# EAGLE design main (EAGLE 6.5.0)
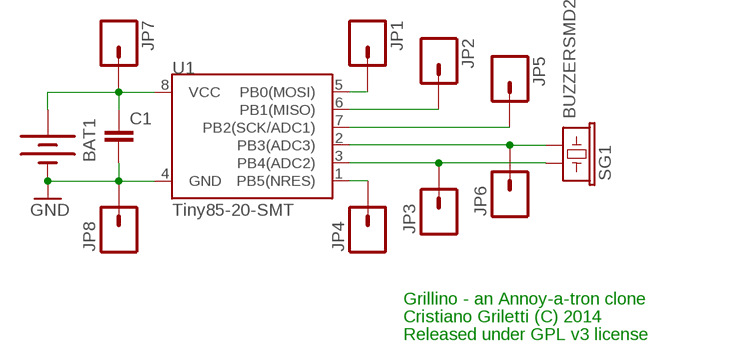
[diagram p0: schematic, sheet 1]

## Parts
BAT1  BATTERYFOB  [BATTERY_20MM_PTH_COMPACT]
C1  CAP0805  [0805]
JP1  M01SMD-4.5X1.5  [PAD-1.5X4.5]
JP2  M01SMD-4.5X1.5  [PAD-1.5X4.5]
JP3  M01SMD-4.5X1.5  [PAD-1.5X4.5]
JP4  M01SMD-4.5X1.5  [PAD-1.5X4.5]
JP5  M01SMD-4.5X1.5  [PAD-1.5X4.5]
JP6  M01SMD-4.5X1.5  [PAD-1.5X4.5]
JP7  M01SMD-4.5X1.5  [PAD-1.5X4.5]
JP8  M01SMD-4.5X1.5  [PAD-1.5X4.5]
SG1  BUZZERSMD2  [BUZZER-CCV]
U1  Tiny85-20-SMT  ATTINY45TINY85-20-SMT  [SO08-EIAJ]

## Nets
GND: BAT1.2(-) C1.2 JP8.P$1 U1.4(GND)
N$2: BAT1.1(+) C1.1 JP7.P$1 U1.8(VCC)
N$3: JP6.P$1 SG1.- U1.2(PB3(ADC3))
N$4: JP5.P$1 U1.7(PB2(SCK/ADC1))
N$5: JP1.P$1 U1.5(PB0(MOSI))
N$6: JP2.P$1 U1.6(PB1(MISO))
N$7: JP3.P$1 SG1.+ U1.3(PB4(ADC2))
N$8: JP4.P$1 U1.1(PB5(NRES))

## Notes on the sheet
- Grillino - an Annoy-a-tron clone
- Cristiano Griletti (C) 2014
- Released under GPL v3 license

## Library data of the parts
BAT1 = SparkFun-Electromechanical:BATTERY: Battery Holders
C1 = SparkFun-Passives:CAP: Capacitor
JP1-JP8 = SparkFun-Connectors:M01: Header 1
SG1 = SparkFun-Electromechanical:BUZZER: Buzzer 12mm
U1 = SparkFun-DigitalIC:ATTINY45: Atmel 8-pin 2/4/8kB flash uC; PROD_ID: IC-09092

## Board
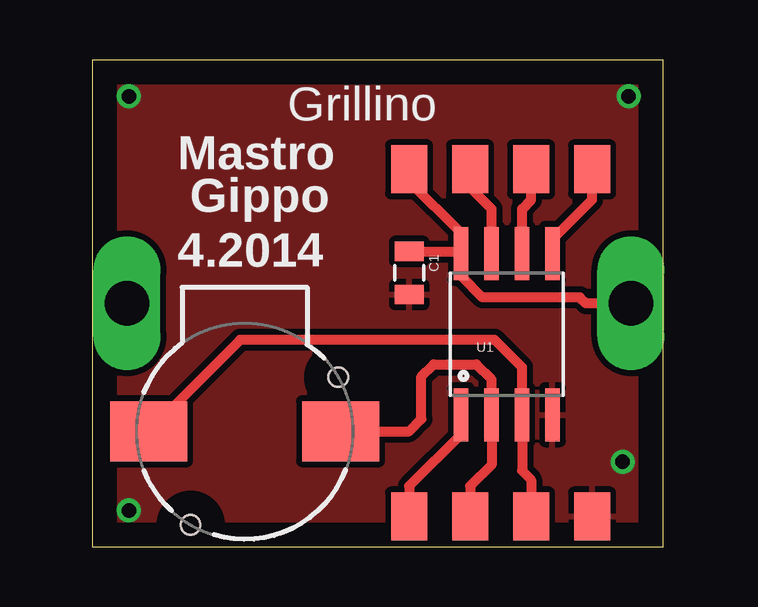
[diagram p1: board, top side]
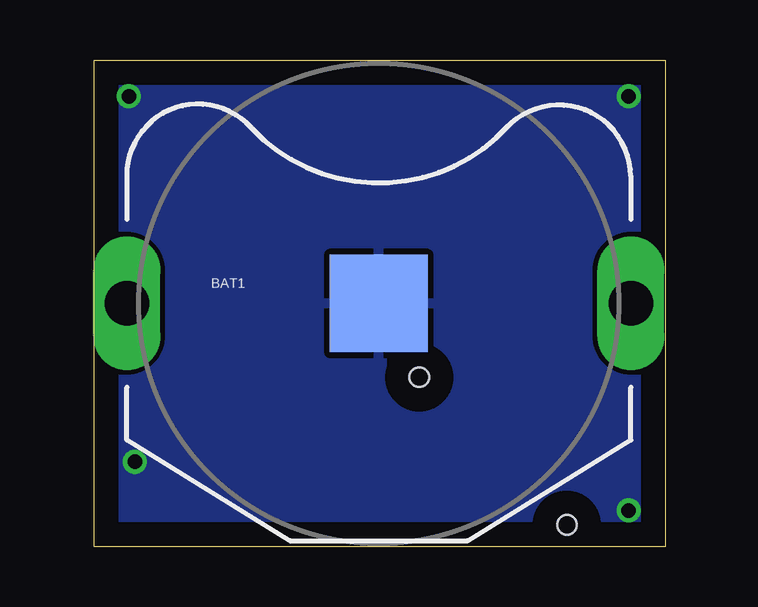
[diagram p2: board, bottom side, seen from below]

Size 23.8 x 20.31 mm. Coordinates in mm from the lower left corner, seen from the top.
Outline: 0,0 23.8,0 23.8,20.31 0,20.31 0,0
Copper layers (1*16): Top 0.035mm / dielectric 1.5mm / Bottom 0.035mm
Design rules "default": minimum track width 10mil, minimum drill 24mil, track to track 8mil, track to pad 8mil, pad to pad 8mil, via to via 8mil, smd to smd 8mil, copper to edge 40mil, drill to drill 8mil, minimum pad ring 10mil, minimum via ring 8mil, stop-mask expansion 4mil, vias tented up to drill 0mil, thermal gap 10mil

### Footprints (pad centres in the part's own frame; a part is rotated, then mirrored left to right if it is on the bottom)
BATTERY_20MM_PTH_COMPACT = drill 1.854 long: 1 -10.5,0; 3 10.5,0 | smd 4.064 x 4.064: 2 0,0
0805 = smd 0.8 x 1.2: 1 -0.9,0; 2 0.9,0
PAD-1.5X4.5 = smd 1.5 x 2: P$1 0,0
BUZZER-CCV = smd 3.2 x 2.5: + 4,0; - -4,0 | hole 0.8: -3.9,-2.25; 2.25,3.9
SO08-EIAJ = smd 0.61 x 2.21: 1 -1.905,-3.378; 2 -0.635,-3.378; 3 0.635,-3.378; 4 1.905,-3.378; 5 1.905,3.353; 6 0.635,3.353; 7 -0.635,3.353; 8 -1.905,3.353

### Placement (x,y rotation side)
BAT1  11.94,10.16 0 bottom
C1  13.21,11.43 270 top
JP1  20.83,15.75 0 top
JP2  18.29,15.75 0 top
JP3  18.29,1.27 0 top
JP4  13.21,1.27 0 top
JP5  15.75,15.75 0 top
JP6  15.75,1.27 0 top
JP7  13.21,15.75 0 top
JP8  20.83,1.27 0 top
SG1  6.35,4.83 180 top
U1  17.27,8.89 0 top

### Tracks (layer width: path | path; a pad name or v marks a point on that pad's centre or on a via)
GND  (via drill 0.6)
  other vias: 1.52,1.52 22.1,3.56 22.35,18.8 1.52,18.8
  pour Bottom: 0,20.32 23.88,20.32 23.88,0 0,0
  pour Top (isolate 0.254): 0,20.32 23.88,20.32 23.88,0 0,0
N$2
  Top 0.406: C1.1 15.28,12.33 U1.8 | JP7.P$1 13.21,15.24 15.37,13.08 U1.8 | BAT1.1 20.57,10.16 20.32,10.41 16.26,10.41 15.37,11.3 U1.8
N$3
  Top 0.406: SG1.- 13.21,4.83 13.72,5.33 13.72,7.11 14.22,7.62 16,7.62 16.64,6.99 U1.2 16.64,3.43 15.75,2.54 JP6.P$1
N$4
  Top 0.406: U1.7 16.64,14.1 15.75,14.99 JP5.P$1
N$5
  Top 0.406: U1.5 19.18,12.83 20.83,14.48 JP1.P$1
N$6
  Top 0.406: U1.6 17.91,14.1 18.29,14.48 JP2.P$1
N$7
  Top 0.406: SG1.+ 6.16,8.64 16.76,8.64 17.91,7.49 U1.3 17.91,3.17 18.29,2.79 JP3.P$1
N$8
  Top 0.406: U1.1 15.37,4.7 13.21,2.54 JP4.P$1

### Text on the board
_tsilk: Grillino | Mastro | Gippo | 4.2014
